(* Logix 5000 AddOnInstructionDefinition export NSL_F_AOI_8P; software revision 33.00 *)

ADD_ON_INSTRUCTION NSL_F_AOI_8P   (* revision 1.0, vendor PM Controls *)
// Anderson-Negele Level Sensor
// Revision note:
// psm
VAR_OUTPUT
   IOLink_Mode : BOOL; {access Read Only, visible}
   Device_Not_Connected : BOOL; {access Read Only, visible}
END_VAR
VAR_IN_OUT
   Input : INT[223]; {required}
END_VAR
VAR_INPUT
   Port_Process_Data_Size : INT := 4;
   Port_Number : INT; {visible}
END_VAR
VAR_OUTPUT
   Vendor_ID : INT; {access Read Only, visible}
   Device_ID : DINT; {access Read Only, visible}
   Invalid_Data : BOOL; {access Read Only, visible}
   Level : REAL; {access Read Only, visible}
   Dry_Run_Detection : REAL; {access Read Only, visible}
END_VAR
VAR
   StatusFlgs_Offset : INT; {access None}
   RealPort_Num : INT; {access None}
   Process_Offset : INT; {access None}
   Offset_StatusFlgs : INT; {access None}
   Offset_Address : INT; {access None}
   Data_Size : INT; {access None}
   LevelDINT : DINT; {access None}
   Dry_Run_Detection_INT : INT[2]; {access None}
   Dry_Run_DetectionDINT : DINT; {access None}
   Level_INT : INT[2]; {access None}
END_VAR

ROUTINE Logic   (* ladder *)
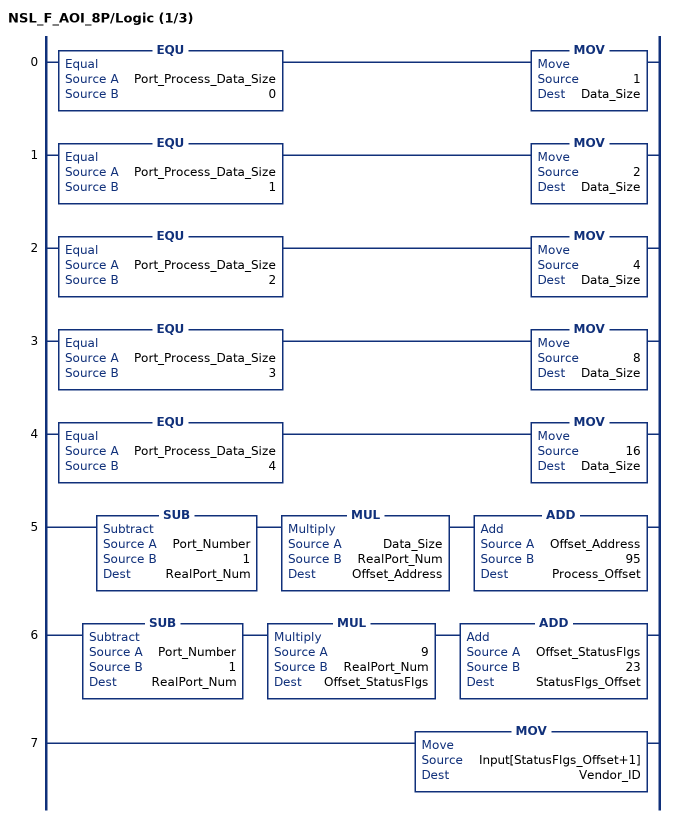
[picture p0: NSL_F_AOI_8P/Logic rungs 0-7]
   0: EQU(Port_Process_Data_Size,0)MOV(1,Data_Size);
   1: EQU(Port_Process_Data_Size,1)MOV(2,Data_Size);
   2: EQU(Port_Process_Data_Size,2)MOV(4,Data_Size);
   3: EQU(Port_Process_Data_Size,3)MOV(8,Data_Size);
   4: EQU(Port_Process_Data_Size,4)MOV(16,Data_Size);
   5: SUB(Port_Number,1,RealPort_Num)MUL(Data_Size,RealPort_Num,Offset_Address)ADD(Offset_Address,95,Process_Offset);
   6: SUB(Port_Number,1,RealPort_Num)MUL(9,RealPort_Num,Offset_StatusFlgs)ADD(Offset_StatusFlgs,23,StatusFlgs_Offset);
   7: MOV(Input[StatusFlgs_Offset+1],Vendor_ID);
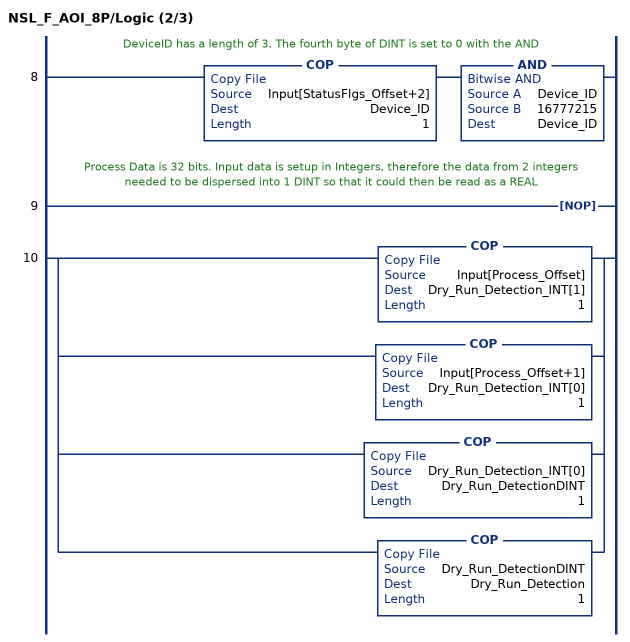
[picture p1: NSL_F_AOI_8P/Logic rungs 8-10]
   // DeviceID has a length of 3. The fourth byte of DINT is set to 0 with the AND
   8: COP(Input[StatusFlgs_Offset+2],Device_ID,1)AND(Device_ID,16777215,Device_ID);
   // Process Data is 32 bits. Input data is setup in Integers, therefore the data from 2 integers needed to be dispersed into 1 DINT so that it could then be read as a REAL
   9: NOP();
   10: [COP(Input[Process_Offset],Dry_Run_Detection_INT[1],1) ,COP(Input[Process_Offset+1],Dry_Run_Detection_INT[0],1) ,COP(Dry_Run_Detection_INT[0],Dry_Run_DetectionDINT,1) ,COP(Dry_Run_DetectionDINT,Dry_Run_Detection,1) ];
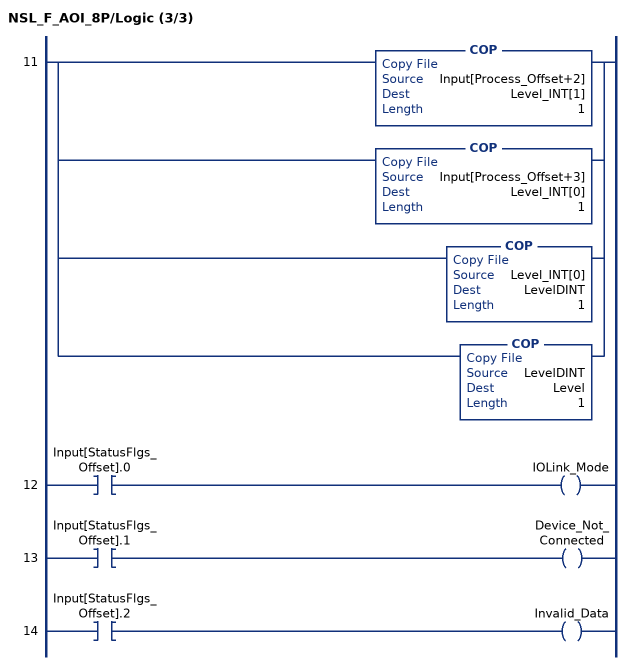
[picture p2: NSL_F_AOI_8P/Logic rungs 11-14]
   11: [COP(Input[Process_Offset+2],Level_INT[1],1) ,COP(Input[Process_Offset+3],Level_INT[0],1) ,COP(Level_INT[0],LevelDINT,1) ,COP(LevelDINT,Level,1) ];
   12: XIC(Input[StatusFlgs_Offset].0)OTE(IOLink_Mode);
   13: XIC(Input[StatusFlgs_Offset].1)OTE(Device_Not_Connected);
   14: XIC(Input[StatusFlgs_Offset].2)OTE(Invalid_Data);
END_ROUTINE
END_ADD_ON_INSTRUCTION
